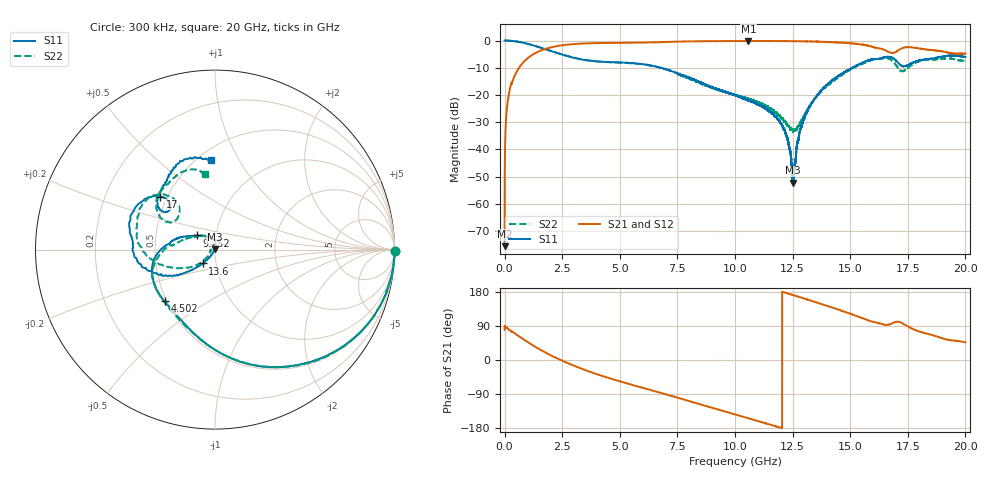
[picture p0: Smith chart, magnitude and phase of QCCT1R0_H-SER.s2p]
!{QCCT1R0}
!Johanson Technology Inc.
!www.johansontechnology.com
!Test Board Conditions:
!Substrate Type  RO4350B
!Substrate Thickness  20 mil
!Substrate Dk  3.66
!TL Type: GCPW
!TL Trace Width  34 mil
!TL Gap  10 mil
!Electrode orientation  Horizontal
!DUT TOPOLOGY	SERIES
!Mounting Pad LxW  26x52 mil
# MHz S  dB  R 50
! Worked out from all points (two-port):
!   20001 points, 300 kHz to 20 GHz, reference 50 ohm
!   highest |S21| = -0.15 dB at 10.58 GHz (marker M1); lowest = -75.6 dB at 300 kHz (marker M2)
!   |S21| within 3 dB of the highest: 1.749 GHz to 16.39 GHz (14.64 GHz wide, 161 % of centre); 17.17 GHz to 18.17 GHz (1.007 GHz wide, 5.7 % of centre)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
!   lowest |S11| = -52.2 dB at 12.51 GHz (marker M3), VSWR 1.00, Z = 49.8 + j0.178 ohm
!   |S11| at or under -10 dB: 6.773984 GHz to 6.774948 GHz (964.3 kHz wide, 0.0142 % of centre); 6.775 GHz to 15.1 GHz (8.325 GHz wide, 76.1 % of centre)
!   |S22| runs from -33.6 to 0.0 dB; largest |S21 - S12| = 0.017
!   S11 on the Smith chart (normalised r, x): 300 kHz: open; 4.502 GHz: 0.49, -0.33; 9.252 GHz: 0.81, +0.13; 13.6 GHz: 0.86, -0.14; 17 GHz: 0.46, +0.33; 20 GHz: 0.58, +0.77
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0.3  0.02 -0.4  -75.59 79.7  -72.00 83.9  0.02 -0.4
101.298  -0.01 -4.8  -24.72 84.8  -24.67 84.9  -0.02 -4.8
134.298  -0.02 -6.3  -22.29 83.3  -22.23 83.2  -0.02 -6.3
517.292  -0.34 -22.0  -11.58 67.0  -11.55 67.1  -0.35 -22.3
1541.277  -2.55 -61.5  -3.79 27.4  -3.77 27.4  -2.55 -61.5
3334.25  -6.93 -111.4  -1.13 -22.8  -1.13 -22.8  -6.90 -112.4
4502.232  -7.92 -134.2  -0.88 -47.2  -0.88 -47.1  -7.95 -138.6
6667.2  -9.76 -175.1  -0.61 -84.9  -0.60 -84.8  -9.80 -172.0
9252.161  -17.94 141.6  -0.21 -130.4  -0.21 -130.5  -18.15 142.9
10000.15  -20.05 130.3  -0.18 -143.5  -0.17 -143.7  -20.06 129.6
10583.14  -21.97 117.5  -0.15 -153.9  -0.20 -153.9  -21.39 123.5
11969.12  -30.22 84.8  -0.19 -178.5  -0.21 -178.6  -27.84 123.9
12247.12  -35.39 82.1  -0.21 176.3  -0.20 176.3  -31.07 135.3
12513.11  -52.21 133.3  -0.21 171.4  -0.24 171.5  -33.13 163.4
12882.11  -31.77 -121.3  -0.25 164.4  -0.27 164.5  -29.37 -149.7
13334.1  -22.77 -127.8  -0.33 155.8  -0.33 155.8  -22.86 -135.6
13595.1  -19.78 -131.1  -0.42 150.7  -0.42 150.7  -19.95 -136.2
15337.07  -9.02 -158.3  -1.26 114.8  -1.26 114.5  -9.20 -169.2
16667.05  -5.97 155.2  -4.19 93.1  -4.39 93.5  -6.57 141.9
17000.04  -7.43 135.9  -4.08 101.0  -4.19 101.2  -9.20 129.2
17615.04  -8.54 144.1  -2.47 84.9  -2.48 84.7  -9.26 150.0
20000  -6.01 92.9  -4.79 46.6  -4.89 46.5  -7.42 97.2
